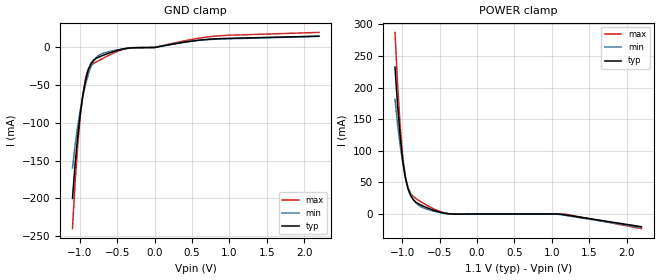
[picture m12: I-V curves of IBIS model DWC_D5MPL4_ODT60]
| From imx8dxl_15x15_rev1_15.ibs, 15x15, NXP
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[Model] DWC_D5MPL4_ODT60
Model_type   Input
Polarity   Non-Inverting
Enable   Active-High
C_comp   1.284pF   1.202pF   1.378pF
C_comp_power_clamp   319.771fF   299.116fF   341.733fF
C_comp_gnd_clamp 947.165fF   886.520fF   1.045pF
Vinh = 640.000mV
Vinl = 460.000mV
[Model Spec]
D_overshoot_ampl_h 0.35 NA   NA
D_overshoot_ampl_l 0.35 NA   NA
D_overshoot_area_l 800.000p NA   NA
D_overshoot_area_h 800.000p NA   NA
[Receiver Thresholds]
Vth = 550.000mV
Vth_min = 539.000mV
Vth_max = 561.000mV
Vinh_ac = 70.000mV
Vinh_dc = 70.000mV
Vinl_ac = -70.000mV
Vinl_dc = -70.000mV
Tslew_ac = 5.000ns
Reference_supply Power_clamp_ref
[Temperature Range]   25.000   125.000   -40.000
[Voltage Range]   1.100V   1.060V   1.170V
[GND Clamp Reference]   0.00V   0.00V   0.00V
[C Comp Corner]
| variable   typ   min   max
C_comp 1.284pF   1.378pF   1.202pF
C_comp_pullup 319.771fF   341.733fF   299.116fF
C_comp_pulldown 947.165fF   1.045pF   886.520fF
[POWER Clamp Reference]   1.100V   1.060V   1.170V
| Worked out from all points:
|   GND clamp passes 1 mA (typ) near -0.36 V on its own axis
|   POWER clamp passes 1 mA (typ) near -0.42 V on its own axis
[GND Clamp]
-1.099V   -200mA     -159.7mA   -240.1mA
-1.064V   -154.9mA   -129.6mA   -179.2mA
-1.028V   -117mA     -103.7mA   -128.9mA
-992.7mV  -86.18mA   -81.72mA   -89.38mA
-957.3mV  -61.73mA   -63.33mA   -59.77mA
-921.8mV  -42.74mA   -47.96mA   -39.39mA
-850.9mV  -20.84mA   -25.3mA    -23.65mA
-744.5mV  -12.6mA    -10.28mA   -17.19mA
-390mV    -1.396mA   -1.485mA   -1.627mA
-1.5uV    -17.22uA   -25.9uA    -13.98uA
815.5mV   11.47mA    10.98mA    15.08mA
2.198V    15.04mA    14.73mA    20mA
[Power Clamp]
-1.098V   232.4mA    181.6mA    287.4mA
-1.063V   172mA      141.7mA    205.1mA
-1.027V   121.1mA    107mA      136.8mA
-991.8mV  82.25mA    78.61mA    87.63mA
-956.4mV  55.67mA    56.97mA    57.38mA
-920.9mV  38.71mA    41.23mA    40.52mA
-850mV    22.08mA    22.46mA    27.29mA
-779.1mV  15.79mA    13.54mA    21.41mA
-708.2mV  11.79mA    9.151mA    16.29mA
-389.1mV  460.3uA    514uA      605uA
1.135V    -634uA     -1.388mA   -10.09uA
2.199V    -20.17mA   -21.32mA   -23.25mA
